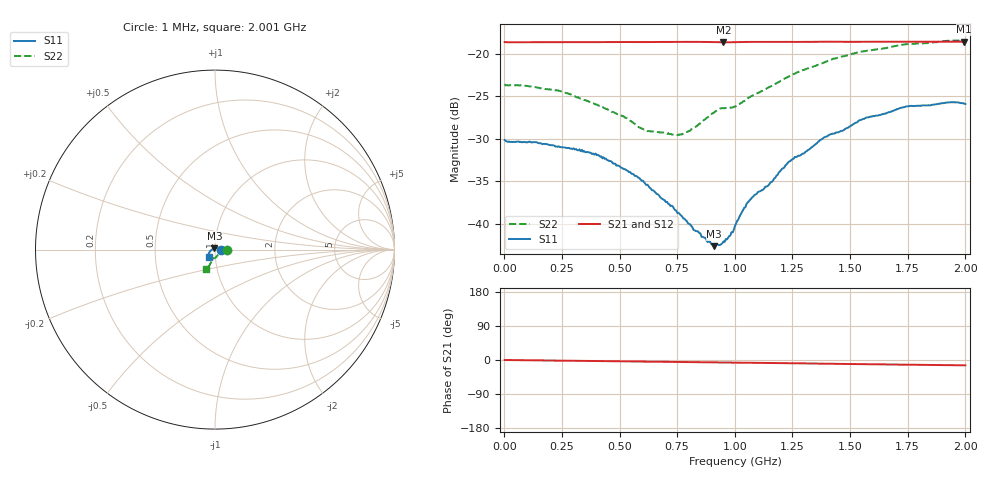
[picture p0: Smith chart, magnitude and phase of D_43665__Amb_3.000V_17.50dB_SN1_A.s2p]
! device id: 43665_
! dir: \\malibu\benchdata\1_engineers\tn_data\43665_75ohm\new\sparar\43665_\amb\3p000v\17p50db
! Serial: 1
! Insertion: A
! Temp: Amb
! VDD: 3.000V
! Attenuation Step: 17.50dB
! IDD: 1.449167e+00mA
! FILE NAME
! DATE 03-27-2009 08:37:38
! CORRECTED  DATA
#  Hz  S  RI  R  75
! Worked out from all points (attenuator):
!   401 points, 1 MHz to 2.001 GHz, reference 75 ohm
!   highest |S21| = -18.53 dB at 1.996 GHz (marker M1); lowest = -18.6 dB at 951 MHz (marker M2)
!   lowest |S11| = -42.6 dB at 911 MHz (marker M3), VSWR 1.01, Z = 74.5 + j0.985 ohm
!   |S11| at or under -10 dB: start of sweep to end of sweep
!   |S22| runs from -29.5 to -18.4 dB; largest |S21 - S12| = 0.00054
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1000000  0.0312 -0.000282  0.1175 -0.000128  0.1177 -0.000204  0.0664 -0.000643
2.36e8  0.028 0.00602  0.1174 -0.00289  0.1175 -0.00286  0.0607 -0.00224
3.36e8  0.0261 0.00781  0.1174 -0.00423  0.1174 -0.00414  0.0542 -0.00427
4.06e8  0.0237 0.00957  0.1174 -0.00505  0.1174 -0.00498  0.0495 -0.00678
5.36e8  0.0177 0.0103  0.1174 -0.00705  0.1175 -0.0069  0.0392 -0.0131
5.96e8  0.0145 0.0106  0.1172 -0.00786  0.1173 -0.0077  0.0326 -0.016
6.71e8  0.0105 0.0103  0.1174 -0.00884  0.1174 -0.0087  0.027 -0.0217
7.76e8  0.00528 0.00942  0.1173 -0.0106  0.1174 -0.0104  0.0169 -0.0295
9.11e8  -0.00332 0.00661  0.1167 -0.013  0.1169 -0.0127  0.00285 -0.0452
9.51e8  -0.00558 0.00559  0.1164 -0.0133  0.1165 -0.013  -0.00428 -0.0479
1.001e9  -0.00836 0.00499  0.1166 -0.0135  0.1167 -0.0133  -0.00896 -0.0482
1.041e9  -0.0118 0.00398  0.1168 -0.0142  0.117 -0.014  -0.011 -0.0516
1.076e9  -0.0142 0.00217  0.1169 -0.015  0.117 -0.0147  -0.0126 -0.0554
1.151e9  -0.0172 -0.000563  0.1166 -0.0161  0.1168 -0.0158  -0.0161 -0.062
1.241e9  -0.0229 -0.00476  0.1165 -0.0176  0.1167 -0.0173  -0.0222 -0.071
1.336e9  -0.0268 -0.00924  0.1164 -0.0189  0.1167 -0.0187  -0.0276 -0.0792
1.386e9  -0.0297 -0.0125  0.1164 -0.0199  0.1168 -0.0197  -0.0287 -0.084
1.546e9  -0.0349 -0.0213  0.1158 -0.0224  0.1163 -0.0223  -0.0378 -0.0959
1.671e9  -0.0363 -0.0274  0.1155 -0.0243  0.1158 -0.0243  -0.0421 -0.1009
1.756e9  -0.0369 -0.0329  0.1153 -0.0255  0.1157 -0.0256  -0.0441 -0.1056
1.996e9  -0.0325 -0.0392  0.1148 -0.0288  0.1148 -0.0291  -0.0507 -0.1084
2.001e9  -0.0326 -0.039  0.1147 -0.0288  0.1147 -0.0291  -0.0509 -0.1083
